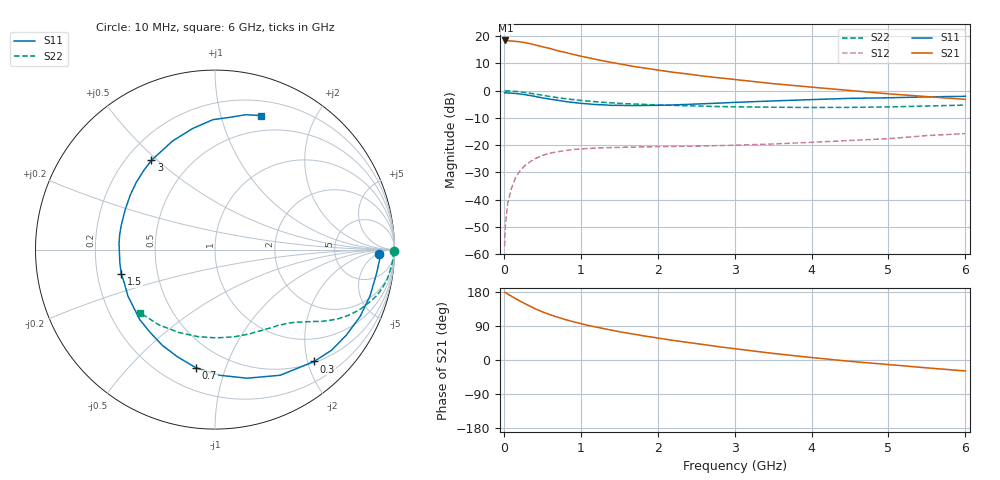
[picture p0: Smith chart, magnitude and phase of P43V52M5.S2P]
! SIEMENS Small Signal Semiconductors
! BFP182
! Si NPN RF Bipolar Junction Transistor in SOT143
! VCE = 3.5 V  IC = 2.5 mA
! Common Emitter S-Parameters:  March  1996
# GHz  S  MA  R  50
!  f  S11  S21  S12  S22
! GHz  MAG  ANG  MAG  ANG  MAG  ANG  MAG  ANG
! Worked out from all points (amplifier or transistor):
!   36 points, 10 MHz to 6 GHz, reference 50 ohm
!   highest |S21| = 18.5 dB at 20 MHz (marker M1)
!   |S21| within 3 dB of that: start of sweep to 606.7 MHz
!   unconditionally stable (mu >= 1): 2.052 GHz to 5.833 GHz
!   at 250 MHz: K = 0.14, MSG = 23.0 dB, |S12| = -28.2 dB
!   at 1.4 GHz: K = 0.73, MSG = 15.6 dB, |S12| = -20.9 dB
!   at 6 GHz: K = 0.98, MSG = 6.3 dB, |S12| = -15.7 dB
!   S11 on the Smith chart (normalised r, x): 10 MHz: 20, -6; 300 MHz: 0.52, -2.12; 700 MHz: 0.33, -0.80; 1.5 GHz: 0.30, -0.12; 3 GHz: 0.30, +0.48; 6 GHz: 0.34, +1.34
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0.01  0.9137 -1.6  8.298 179.0  0.0014 89.5  0.9952 -0.6
0.02  0.9196 -3.3  8.37 178.1  0.0034 80.6  0.9935 -1.3
0.05  0.9096 -8.6  8.291 174.1  0.0086 87.9  0.9927 -3.3
0.1  0.9016 -16.6  8.174 168.2  0.0164 79.5  0.9834 -6.5
0.2  0.8732 -33.1  7.927 156.5  0.0323 71.3  0.9577 -12.8
0.25  0.8579 -40.8  7.737 151.0  0.0389 66.8  0.9388 -15.6
0.3  0.833 -48.4  7.527 146.2  0.0454 63.5  0.9152 -18.2
0.4  0.7891 -62.5  6.97 136.0  0.0562 56.0  0.8717 -22.7
0.5  0.7385 -76.0  6.414 127.2  0.0647 49.6  0.8264 -26.4
0.6  0.7007 -87.9  5.963 119.6  0.0713 44.4  0.7832 -29.6
0.7  0.6673 -99.1  5.428 113.0  0.0758 40.2  0.7455 -32.0
0.8  0.6335 -109.1  5.033 106.6  0.0796 36.2  0.7137 -34.1
0.9  0.6089 -118.8  4.652 101.3  0.0835 33.3  0.6873 -35.6
1.1  0.5726 -137.0  4.038 91.0  0.0873 28.5  0.6446 -38.7
1.5  0.5394 -165.5  3.117 74.7  0.091 22.6  0.5868 -44.0
1.8  0.536 175.9  2.647 64.3  0.0931 20.4  0.5631 -47.7
2.2  0.5474 156.3  2.183 51.8  0.0947 18.5  0.5393 -53.5
3  0.6107 125.5  1.608 29.8  0.1 18.7  0.5079 -67.4
3.5  0.6498 111.3  1.349 17.4  0.1053 19.0  0.4976 -77.5
4.5  0.7243 90.8  1.009 -3.5  0.1222 19.6  0.4943 -101.4
5.5  0.7705 77.2  0.78 -20.8  0.1501 18.3  0.5237 -127.1
6  0.7894 71.1  0.693 -28.9  0.1634 15.0  0.545 -139.7
